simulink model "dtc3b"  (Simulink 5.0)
settings: Solver=ode23  StartTime=0.0  StopTime=2  MaxStep=3e-6  RelTol=1e-3
InitFcn:
  | warning off; wmo=0.0%initial speed
  | fso=1.0 %initial stator flux
  | Vdc=1.0 %
undefined symbols (not defined in the file or in its folder): a, wmo
libraries: simulink x3

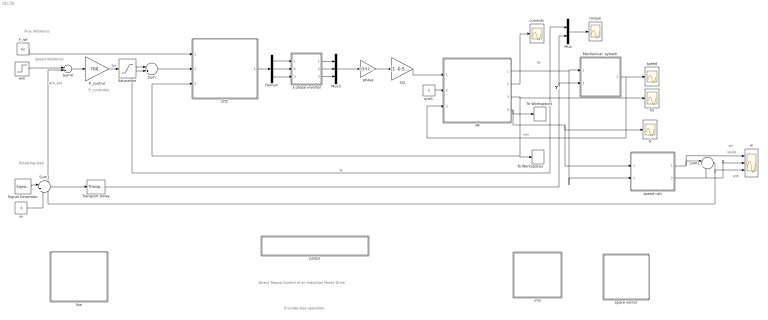
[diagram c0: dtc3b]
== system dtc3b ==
  note: Direct Torque Control of an Induction Motor Drive
  note: Flux reference
  note: Speed reference
  note: Te
  note: Tl
  note: Pulsating load
  note: P_controller
  note: Encoder-less operation
  note: wr
  note: wslip
  note: wm
  note: wm_est
  3 phase inverter : Subsystem
  3/2 : Gain  Gain=[1 -0.5 -0.5;0 sqrt(3)/2 -sqrt(3)/2]  Multiplication=Matrix(K*u)
  DTC : Subsystem
  Demux : Demux  Outputs=3
  F_ref : Constant  Value=fso
  IM : Subsystem  mask{Rs=0.01, Rr=0.02, Lsl=0.10, Lrl=0.10, Lm=4.5, wo=2*pi*60}
      mask prompts: Rs "Stator resistance [pu]"; Rr "Rotor resistance [pu]"; Lsl "Stator leakage inductance [pu]"; Lrl "Rotor leakage inductance [pu]"; Lm "Magnetizing inductance [pu]"; wo "Base frequency [rad/s]"
  Mechanical  system : Subsystem  mask{H=0.5, Bm=1e-5}
      mask prompts: H "Inertia constant [s]"; Bm "Torque-speed coefficient"
  Mux : Mux  Inputs=2
  Mux3 : Mux  Inputs=3
  P_control : Gain  Gain=700
  Saturation : Saturate  UpperLimit=2  LowerLimit=-2
  Signal Generator : SignalGenerator  WaveForm=square  Amplitude=.5  Frequency=4
  Sum : Sum  Inputs=|+-
  Sum1 : Sum  Inputs=|++
  Sum2 : Sum  Inputs=|+-
  Sum4 : Sum  Inputs=|+-
  To Workspace1 : ToWorkspace  VariableName=fr  SampleTime=-1  SaveFormat=Array
  To Workspace2 : ToWorkspace  VariableName=fs  SampleTime=-1  SaveFormat=Array
  Transport Delay : TransportDelay
  currents : Scope
  fr : Scope
  frs : Scope
  fsw : Subsystem
  info : Subsystem
  one1 : Constant  Value=0
  phase : Gain  Gain=1/3*[2 -1 -1;-1 2 -1;-1 -1 2]  Multiplication=Matrix(K*u)
  plots2 : Subsystem
  space vector : Subsystem
  speed : Scope
  speed calc : Subsystem
  torque : Scope
  w : Scope  NumInputPorts=3
  wm : Step  Time=.2  Before=wmo  After=.8  SampleTime=0
  xx : Constant  Value=.5
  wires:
  F_ref/1 -> DTC/1(f_ref)
  3/2/1 -> IM/1(vs)
  IM/3(fs) -> To Workspace2/1, DTC/3(fs), frs/1
  one1/1 -> IM/2(wk)
  IM/1(Te) -> Mux/1, Mechanical  system/1(Te), speed calc/2(Te), Sum/2  "Te"
  Mechanical  system/1(wm) -> speed/1, IM/3(wm)  "wm"
  IM/2(is) -> currents/1
  wm/1 -> Sum4/1
  Sum/1 -> DTC/2(T_er)
  Mux/1 -> torque/1
  Sum4/1 -> P_control/1
  P_control/1 -> Saturation/1  "Te*"
  IM/4(fr) -> To Workspace1/1, fr/1, speed calc/1(fr)
  Signal Generator/1 -> Sum1/1
  xx/1 -> Sum1/2
  Sum1/1 -> Transport Delay/1
  Transport Delay/1 -> Mux/2, Mechanical  system/2(Tl)
  Saturation/1 -> Sum/1
  speed calc/1(wr) -> Sum2/1, w/1
  speed calc/2(wslip) -> Sum2/2, w/2
  Sum2/1 -> w/3, Sum4/2
  Mux3/1 -> phase/1
  Demux/1 -> 3 phase inverter/1(sa)
  Demux/2 -> 3 phase inverter/2(sb)
  Demux/3 -> 3 phase inverter/3(sc)
  3 phase inverter/1(va) -> Mux3/1
  3 phase inverter/2(vb) -> Mux3/2
  3 phase inverter/3(vc) -> Mux3/3
  DTC/1(s3) -> Demux/1
  phase/1 -> 3/2/1

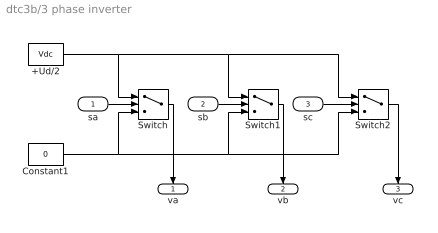
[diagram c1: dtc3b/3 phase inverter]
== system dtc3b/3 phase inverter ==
  sa : Inport
  sb : Inport  Port=2
  sc : Inport  Port=3
  +Ud/2 : Constant  Value=Vdc
  Constant1 : Constant  Value=0
  Switch : Switch  Threshold=0.5
  Switch1 : Switch  Threshold=0.5
  Switch2 : Switch  Threshold=0.5
  va : Outport  Orientation=down  InitialOutput=0
  vb : Outport  Orientation=down  Port=2  InitialOutput=0
  vc : Outport  Orientation=down  Port=3  InitialOutput=0
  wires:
  Switch1/1 -> vb/1
  Switch2/1 -> vc/1
  sc/1 -> Switch2/2
  sb/1 -> Switch1/2
  Switch/1 -> va/1
  sa/1 -> Switch/2
  Constant1/1 -> Switch2/3, Switch1/3, Switch/3
  +Ud/2/1 -> Switch2/1, Switch1/1, Switch/1

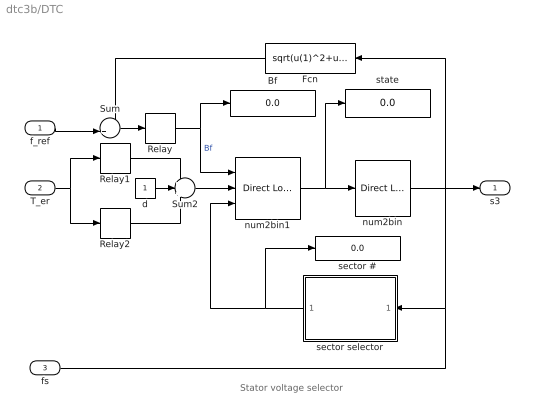
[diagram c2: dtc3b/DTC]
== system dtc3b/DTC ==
  note: Stator voltage selector
  f_ref : Inport
  T_er : Inport  Port=2
  fs : Inport  Port=3
  Bf : Display
  Fcn : Fcn  Orientation=left  Expr=sqrt(u(1)^2+u(2)^2)
  Relay : Relay  OnSwitchValue=.01  OffSwitchValue=-.01
  Relay1 : Relay  OnSwitchValue=.02  OffSwitchValue=0
  Relay2 : Relay  OnSwitchValue=0  OffSwitchValue=-.02  OnOutputValue=0  OffOutputValue=-1
  Sum : Sum  Inputs=-+|
  Sum2 : Sum  Inputs=+++
  d : Constant
  num2bin : simulink/Look-Up Tables/Direct Look-Up Table (n-D)  maskTabDims=2  explicitNumDims=1  outDims=Column  tabIsInput=off  mxTable=[0 0 0;1 0 0;0 1 0;1 1 0;0 0 1;1 0 1;0 1 1;1 1 1]'  clipFlag=Error
  num2bin1 : simulink/Look-Up Tables/Direct Look-Up Table (n-D)  maskTabDims=3  explicitNumDims=1  outDims=Element  tabIsInput=off  mxTable=a  clipFlag=Error
  sector # : Display
  sector selector : Subsystem  Orientation=left
  state : Display
  s3 : Outport
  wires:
  num2bin1/1 -> state/1, num2bin/1
  Sum/1 -> Relay/1
  Relay/1 -> Bf/1, num2bin1/1  "Bf"
  Fcn/1 -> Sum/1
  Sum2/1 -> num2bin1/2
  Relay1/1 -> Sum2/1
  Relay2/1 -> Sum2/3
  d/1 -> Sum2/2
  T_er/1 -> Relay2/1, Relay1/1
  f_ref/1 -> Sum/2
  num2bin/1 -> s3/1
  fs/1 -> Fcn/1, sector selector/1(fs)
  sector selector/1(sector) -> num2bin1/3, sector #/1

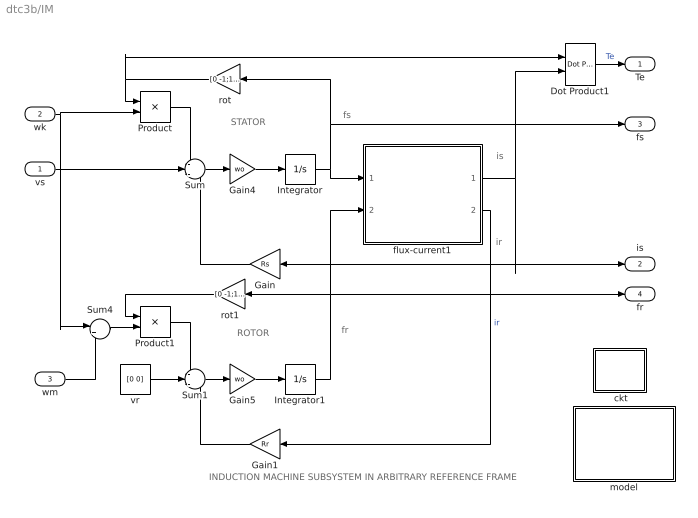
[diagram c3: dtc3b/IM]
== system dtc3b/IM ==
  note: ROTOR
  note: STATOR
  note: fs
  note: fr
  note: is
  note: INDUCTION MACHINE SUBSYSTEM IN ARBITRARY REFERENCE FRAME
  note: ir
  vs : Inport
  wk : Inport  Port=2
  wm : Inport  Port=3
  " ckt" : Subsystem
  Dot Product1 : simulink/Math Operations/Dot Product
  Gain : Gain  Orientation=left  Gain=Rs
  Gain1 : Gain  Orientation=left  Gain=Rr
  Gain4 : Gain  Gain=wo
  Gain5 : Gain  Gain=wo
  Integrator : Integrator  InitialCondition=[fso 0]
  Integrator1 : Integrator  InitialCondition=[fso 0]
  Product : Product
  Product1 : Product
  Sum : Sum  Inputs=-+-
  Sum1 : Sum  Inputs=-+-
  Sum4 : Sum  Inputs=|+-
  flux-current1 : Subsystem
  model : Subsystem
  rot : Gain  Orientation=left  Gain=[0 -1;1 0]  Multiplication=Matrix(K*u)
  rot1 : Gain  Orientation=left  Gain=[0 -1;1 0]  Multiplication=Matrix(K*u)
  vr : Constant  Value=[0 0]
  Te : Outport
  is : Outport  Port=2
  fs : Outport  Port=3
  fr : Outport  Port=4
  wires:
  Gain/1 -> Sum/3
  vr/1 -> Sum1/2
  Gain1/1 -> Sum1/3
  flux-current1/2(ir) -> Gain1/1  "ir"
  Integrator/1 -> flux-current1/1(fs), rot/1, fs/1
  Integrator1/1 -> flux-current1/2(fr), rot1/1, fr/1
  Product1/1 -> Sum1/1
  rot1/1 -> Product1/1
  Product/1 -> Sum/1
  rot/1 -> Product/1, Dot Product1/1
  Sum4/1 -> Product1/2
  Sum/1 -> Gain4/1
  Gain4/1 -> Integrator/1
  Sum1/1 -> Gain5/1
  Gain5/1 -> Integrator1/1
  flux-current1/1(is) -> Gain/1, is/1, Dot Product1/2
  Dot Product1/1 -> Te/1  "Te"
  vs/1 -> Sum/2
  wk/1 -> Product/2, Sum4/1
  wm/1 -> Sum4/2

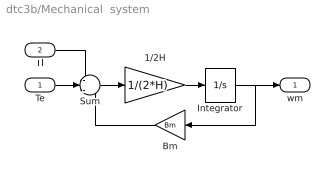
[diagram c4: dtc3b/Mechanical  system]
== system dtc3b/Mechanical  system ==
  Te : Inport
  Tl : Inport  Port=2
  1/2H : Gain  Gain=1/(2*H)
  Bm : Gain  Orientation=left  Gain=Bm
  Integrator : Integrator  InitialCondition=wmo
  Sum : Sum  Inputs=-+-
  wm : Outport
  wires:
  Tl/1 -> Sum/1
  Te/1 -> Sum/2
  Integrator/1 -> wm/1, Bm/1
  Bm/1 -> Sum/3
  Sum/1 -> 1/2H/1
  1/2H/1 -> Integrator/1

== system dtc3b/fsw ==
  note: Script files
  note: This collection of demonstrations is designed to illustrate the use of MATLAB for the simulation of the steady-state characteristics of ac machines under balanced and unbalanced conditions of operation.

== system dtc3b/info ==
  note: Direct torque control of an induction motordrive
  note: The induction motor operates initially at no load at a speed and a stator flux level specified in a callback of the model properties. The mechanical load torque is initially set at Tl = 0 and the electromagnetic torque Te is set to zero by having stator and rotor space vectors colinear (check the IC's of the flux integrators). Before running, double click the Switching Table block.

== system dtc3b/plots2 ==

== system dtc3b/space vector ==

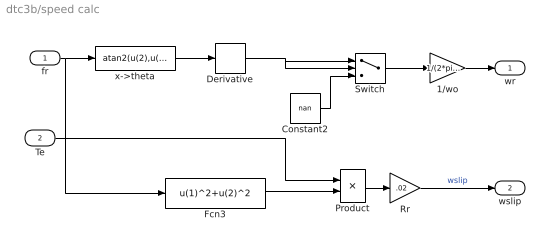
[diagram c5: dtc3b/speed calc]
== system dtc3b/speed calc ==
  fr : Inport
  Te : Inport  Port=2
  1/wo : Gain  Gain=1/(2*pi*60)
  Constant2 : Constant  Value=nan
  Derivative : Derivative
  Fcn3 : Fcn  Expr=u(1)^2+u(2)^2
  Product : Product  Inputs=*/
  Rr : Gain  Gain=.02
  Switch : Switch
  x->theta : Fcn  Expr=atan2(u(2),u(1))
  wr : Outport
  wslip : Outport  Port=2
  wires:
  Switch/1 -> 1/wo/1
  Constant2/1 -> Switch/3
  Derivative/1 -> Switch/1, Switch/2
  fr/1 -> x->theta/1, Fcn3/1
  1/wo/1 -> wr/1
  x->theta/1 -> Derivative/1
  Fcn3/1 -> Product/2
  Product/1 -> Rr/1
  Te/1 -> Product/1
  Rr/1 -> wslip/1  "wslip"

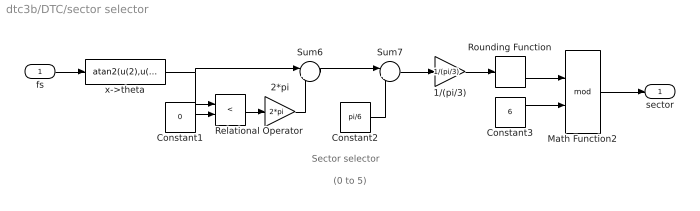
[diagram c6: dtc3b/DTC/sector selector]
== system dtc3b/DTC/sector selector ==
  note: Sector selector
  note: (0 to 5)
  fs : Inport
  1/(pi/3) : Gain  Gain=1/(pi/3)
  2*pi : Gain  Gain=2*pi
  Constant1 : Constant  Value=0
  Constant2 : Constant  Value=pi/6
  Constant3 : Constant  Value=6
  Math Function2 : Math  Operator=mod
  Relational Operator : RelationalOperator  Operator=<
  Rounding Function : Rounding
  Sum6 : Sum  Inputs=|++
  Sum7 : Sum  Inputs=|++
  x->theta : Fcn  Expr=atan2(u(2),u(1))
  sector : Outport
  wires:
  Constant1/1 -> Relational Operator/2
  Relational Operator/1 -> 2*pi/1
  2*pi/1 -> Sum6/2
  Sum6/1 -> Sum7/1
  Constant2/1 -> Sum7/2
  Sum7/1 -> 1/(pi/3)/1
  1/(pi/3)/1 -> Rounding Function/1
  Rounding Function/1 -> Math Function2/1
  Constant3/1 -> Math Function2/2
  fs/1 -> x->theta/1
  Math Function2/1 -> sector/1
  x->theta/1 -> Relational Operator/1, Sum6/1

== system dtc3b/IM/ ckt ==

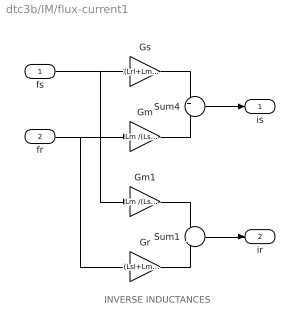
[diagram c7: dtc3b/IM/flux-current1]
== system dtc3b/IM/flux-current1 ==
  note: INVERSE INDUCTANCES
  fs : Inport
  fr : Inport  Port=2
  Gm : Gain  Gain=Lm /(Lsl*Lrl+Lsl*Lm+Lrl*Lm)
  Gm1 : Gain  Gain=Lm /(Lsl*Lrl+Lsl*Lm+Lrl*Lm)
  Gr : Gain  Gain=(Lsl+Lm )/(Lsl*Lrl+Lsl*Lm+Lrl*Lm)
  Gs : Gain  Gain=(Lrl+Lm) /(Lsl*Lrl+Lsl*Lm+Lrl*Lm)
  Sum1 : Sum  Inputs=-+
  Sum4 : Sum  Inputs=+-
  is : Outport
  ir : Outport  Port=2
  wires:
  fs/1 -> Gs/1, Gm1/1
  Gs/1 -> Sum4/1
  fr/1 -> Gm/1, Gr/1
  Gm/1 -> Sum4/2
  Sum4/1 -> is/1
  Gm1/1 -> Sum1/1
  Gr/1 -> Sum1/2
  Sum1/1 -> ir/1

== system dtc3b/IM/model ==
  note: Mathematical model of the induction machine. State vector formulation in an arbitrary dq common reference frame. Per unit description.
  note: Electrical system equations: vs = Rs is + 1/wo (dfs/dt) + wk M(pi/2) fs vr = Rr ir + 1/wo (dfr/dt) + (wk - wm) M(pi/2) fr where the variables i, v, and f are 2-dimensional space vectors; for instance is = [ids iqs] and so forth, wk is the speed of the reference frame, wm the rotor speed, and M(pi/2)represents a 90o space rotator namely M(pi/2) = [0 -1;1 0] The flux linkage current relations are: fds = Ls ids + Lm idr fdr = Lm ids + Lr idr (D_axis) Ls =Lm +Lsl ; Lr = Lm +Lrl fqs = Ls iqs + Lm iqr fqr = Lm iqs + Lr iqr (Q_axis) Mechanical system equations: Te = 2H (dwm/dt ) + Bm wm + Tl where Te = fs (cross) is = M(pi/2) fs (dot) is = fds iqs - fqs ids = fs x is = M(pi/2) fs . is = ir x fr = Lm (ir x is) = Lm/Lr (fr x is) = 1/Lm' (fr x fs) Lm' =Lm c/(1-c) c = 1 - Lm^2/(Ls Lr)
